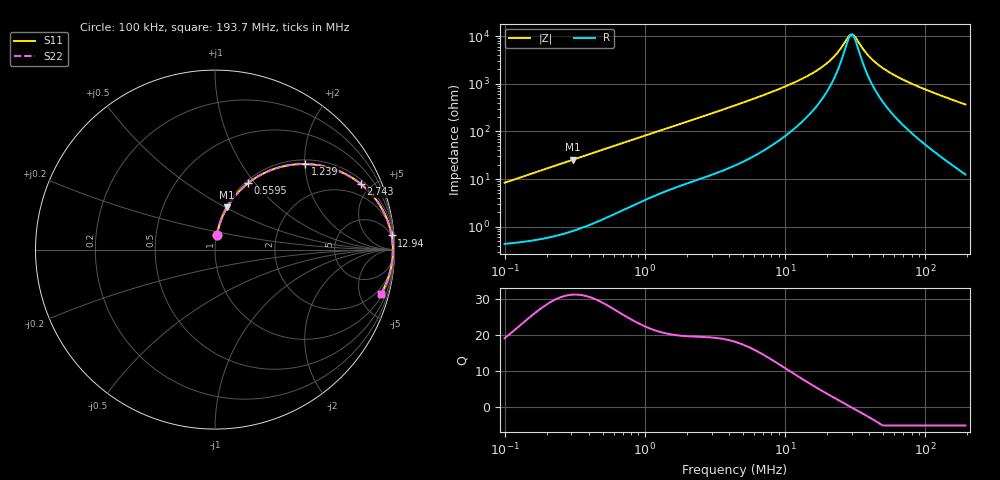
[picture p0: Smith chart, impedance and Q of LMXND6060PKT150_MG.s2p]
! LMXND6060PKT150_MG  S-PARAMETER MODEL  ( General Type )
! Model Generated by TAIYO YUDEN Corporation (https://www.yuden.co.jp/en/)
! Version 1.0
! TAIYO YUDEN Control No. 191025NI43SB-FBB
! Copyright(c) 2019 TAIYO YUDEN CO.,LTD. All Rights Reserved.
! Product Description (link to TY-COMPAS)
! https://ds.yuden.co.jp/TYCOMPAS/or/detail?pn=LMXND6060PKT150MMG&u=M
! Products Name : Inductors
! Characteristics :
!  Inductance : 15 uH , SRF(min) : 20 MHz , DC Resistance(max) : 0.252 Ohm
!  Rated Current : Saturation :1150 mA , Temp Rise : 1200 mA (40 degC)
!  Case Size : 6.0 x 6.0 / 0.236 x 0.236 [mm/inch] , Thickness : 1.4 / 0.055 [mm/inch]
!  (Conditions: Temperature = 25 degC , DC Bias Current/Voltage = 0A / 0V)
! External Node Assignments :
!  1  o---GGG---o  2
! GND o---------o GND
! Frequency Range : 0.1MHz  -  193.730505MHz  [ 402 STEP ]
# MHz S RI R 50
! Freq[MHz].  S11 Real  S11 Imag  S21 Real  S21 Imag  S12 Real  S12 Imag  S22 Real  S22 Imag
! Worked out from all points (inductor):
!   401 points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, 100 kHz to 193.7 MHz, reference 50 ohm
!   read as one part in series: L = 13.3 uH near 103.9 kHz
!   highest Q = 31.3 at 305.4 kHz (marker M1), where L = 13.2 uH
!   self-resonance near 29.76 MHz
!   S11 on the Smith chart (normalised r, x): 100 kHz: 1.01, +0.17; 559.5 kHz: 1.03, +0.92; 1.239 MHz: 1.09, +2.01; 2.743 MHz: 1.22, +4.35; 12.94 MHz: 4, +24; 193.7 MHz: 1.25, -7.34
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0.1  0.0112 0.0825  0.9888 -0.0825  0.9888 -0.0825  0.0112 0.0825
0.305395  0.0671 0.2347  0.9329 -0.2347  0.9329 -0.2347  0.0671 0.2347
0.355309  0.0872 0.2665  0.9128 -0.2665  0.9128 -0.2665  0.0872 0.2665
0.559548  0.1845 0.3704  0.8155 -0.3704  0.8155 -0.3704  0.1845 0.3704
0.864672  0.3401 0.4531  0.6599 -0.4531  0.6599 -0.4531  0.3401 0.4531
1.238778  0.5018 0.4769  0.4982 -0.4769  0.4982 -0.4769  0.5018 0.4769
1.262442  0.5106 0.4767  0.4894 -0.4767  0.4894 -0.4767  0.5106 0.4767
2.742516  0.814 0.3643  0.186 -0.3643  0.186 -0.3643  0.814 0.3643
4.401483  0.9131 0.2555  0.0869 -0.2555  0.0869 -0.2555  0.9131 0.2555
8.064452  0.9683 0.1415  0.0317 -0.1415  0.0317 -0.1415  0.9683 0.1415
12.9427  0.9839 0.0787  0.0161 -0.0787  0.0161 -0.0787  0.9839 0.0787
15.63884  0.987 0.0585  0.013 -0.0585  0.013 -0.0585  0.987 0.0585
21.573  0.9899 0.0281  0.0101 -0.0281  0.0101 -0.0281  0.9899 0.0281
24.16677  0.9904 0.0182  0.00957 -0.0182  0.00957 -0.0182  0.9904 0.0182
28.11658  0.9908 0.00526  0.00921 -0.00526  0.00921 -0.00526  0.9908 0.00526
29.75887  0.9908 0.000459  0.00916 -0.000459  0.00916 -0.000459  0.9908 0.000459
31.49709  0.9908 -0.00434  0.00916 0.00434  0.00916 0.00434  0.9908 -0.00434
37.345  0.9905 -0.0189  0.00947 0.0189  0.00947 0.0189  0.9905 -0.0189
41.83506  0.9901 -0.0288  0.00993 0.0288  0.00993 0.0288  0.9901 -0.0288
55.56615  0.9878 -0.0556  0.0122 0.0556  0.0122 0.0556  0.9878 -0.0556
92.61817  0.9773 -0.1156  0.0227 0.1156  0.0227 0.1156  0.9773 -0.1156
193.7305  0.9237 -0.249  0.0763 0.249  0.0763 0.249  0.9237 -0.249
